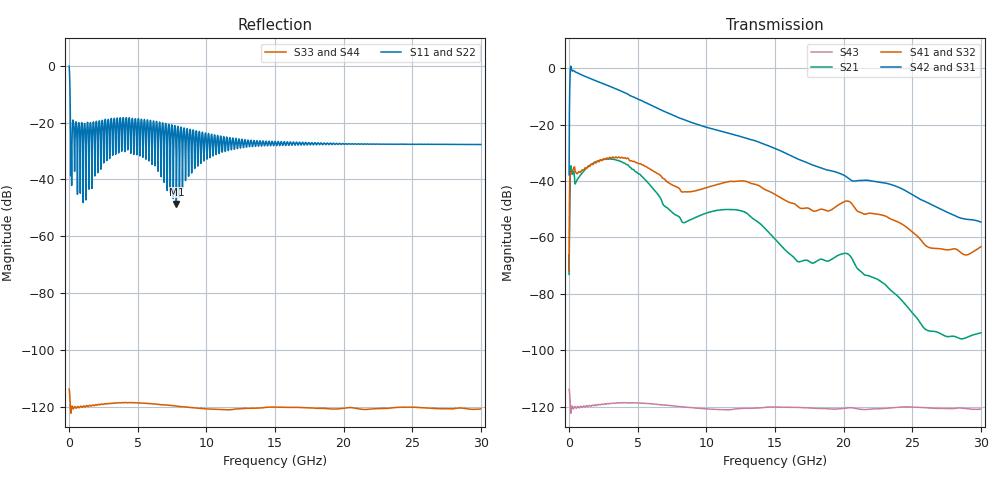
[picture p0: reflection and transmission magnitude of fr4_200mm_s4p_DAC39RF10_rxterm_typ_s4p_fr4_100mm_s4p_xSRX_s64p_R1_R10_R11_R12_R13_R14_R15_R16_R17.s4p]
! Touchstone generated by fitter/viewer
# HZ S  RI R 5.000000e+01
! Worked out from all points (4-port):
!   3899 points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, 7.694 MHz to 30 GHz, reference 50 ohm
!   strongest paths, dB at 7.694 MHz, 7.502 GHz, 15 GHz, 22.51 GHz, 30 GHz:
!     S42: -37.8, -16.5, -28.5, -40.4, -54.6
!     S31: -37.8, -16.6, -28.5, -40.5, -54.7
!     S41: -71.7, -41.4, -44.7, -51.7, -63.3
!     S32: -71.5, -41.4, -44.9, -51.7, -63.1
!     S21: -73.1, -51.1, -60.6, -74.9, -93.8
!     S43: -113.8, -119.6, -120.1, -120.7, -120.8
!   lowest |S11| = -48.6 dB at 7.817 GHz (marker M1), VSWR 1.01, Z = 49.9 + j0.353 ohm
!   |S11| at or under -10 dB: 76.78 MHz to end of sweep
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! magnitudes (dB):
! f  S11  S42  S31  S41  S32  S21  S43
! 7.694 MHz  -0.1  -37.8  -37.8  -71.7  -71.5  -73.1  -113.8
! 223.1 MHz  -25.6  -0.9  -0.9  -36.2  -36.3  -37.5  -119.7
! 2.439 GHz  -19.4  -5.4  -5.4  -32.6  -32.6  -32.4  -119.2
! 7.817 GHz  -48.6  -17.1  -17.2  -42.0  -42.0  -52.1  -119.8
! 12.67 GHz  -28.0  -24.5  -24.5  -40.0  -40.2  -50.8  -120.6
! 23.81 GHz  -27.6  -41.8  -41.9  -54.2  -54.4  -80.2  -120.2
! 30 GHz  -27.7  -54.6  -54.7  -63.3  -63.1  -93.8  -120.8
